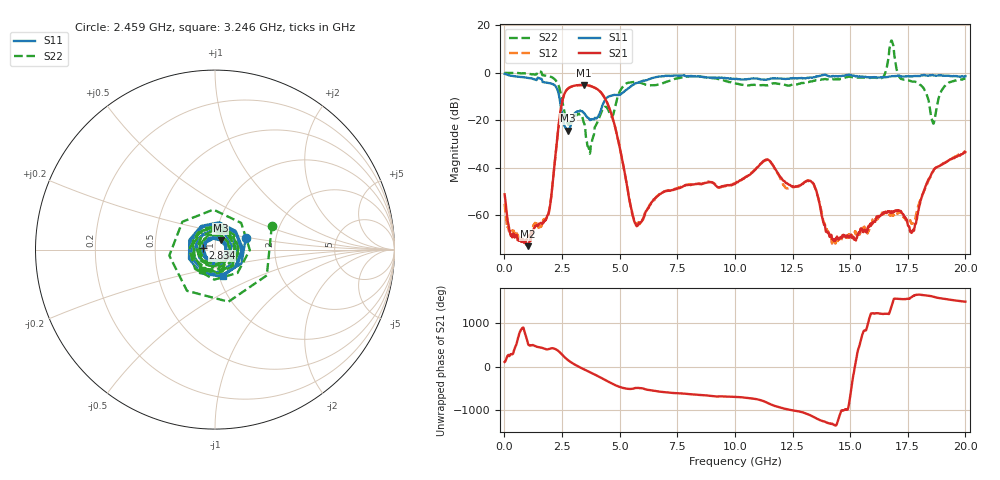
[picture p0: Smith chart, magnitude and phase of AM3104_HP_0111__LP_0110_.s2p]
!Created with skrf (http://scikit-rf.org).
# Hz S RI R 50.0
!freq ReS11 ImS11 ReS21 ImS21 ReS12 ImS12 ReS22 ImS22
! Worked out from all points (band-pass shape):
!   1601 points, 10 MHz to 20 GHz, reference 50 ohm
!   highest |S21| = -5.14 dB at 3.433 GHz (marker M1); lowest = -73.1 dB at 1.01 GHz (marker M2)
!   |S21| within 3 dB of the highest: 2.642 GHz to 4.179 GHz (1.537 GHz wide, 45.1 % of centre)
!   lowest |S11| = -24.4 dB at 2.759 GHz (marker M3), VSWR 1.13, Z = 53 + j5.47 ohm
!   |S11| at or under -10 dB: 2.38 GHz to 4.522 GHz (2.141 GHz wide, 62.1 % of centre)
!   |S22| runs from -34.1 to 13.6 dB; largest |S21 - S12| = 0.03
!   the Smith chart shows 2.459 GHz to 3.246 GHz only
!   S11 on the Smith chart (normalised r, x): 2.459 GHz: 1.40, +0.19; 2.834 GHz: 0.87, +0.02; 3.246 GHz: 1.05, -0.31
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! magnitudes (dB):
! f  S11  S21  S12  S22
! 10 MHz  -0.4  -51.3  -55.3  0.0
! 284.9 MHz  -1.2  -68.5  -67.4  -0.1
! 1.01 GHz  -2.1  -73.1  -70.2  -0.4
! 1.909 GHz  -4.3  -59.5  -59.8  -1.4
! 2.459 GHz  -14.8  -14.7  -14.8  -9.3
! 2.759 GHz  -24.4  -6.7  -6.7  -21.6
! 2.834 GHz  -23.2  -6.1  -6.2  -21.5
! 3.246 GHz  -16.3  -5.1  -5.2  -17.5
! 3.346 GHz  -16.2  -5.2  -5.2  -17.8
! 3.433 GHz  -16.8  -5.1  -5.2  -20.7
! 3.696 GHz  -19.7  -5.5  -5.5  -34.0
! 4.545 GHz  -9.9  -14.7  -14.8  -16.7
! 5.707 GHz  -4.5  -64.2  -63.5  -3.8
! 6.682 GHz  -1.6  -51.8  -51.5  -5.0
! 10.01 GHz  -2.7  -46.9  -46.6  -4.5
! 11.38 GHz  -2.9  -36.6  -36.8  -5.3
! 13.34 GHz  -2.1  -46.2  -46.0  -3.6
! 14.29 GHz  -1.4  -70.3  -71.1  -2.8
! 16.68 GHz  -1.6  -58.7  -59.6  7.2
! 17.7 GHz  -1.5  -67.1  -63.7  -3.7
! 18.6 GHz  -1.1  -41.5  -41.6  -21.3
! 20 GHz  -1.5  -33.5  -33.1  -2.5
